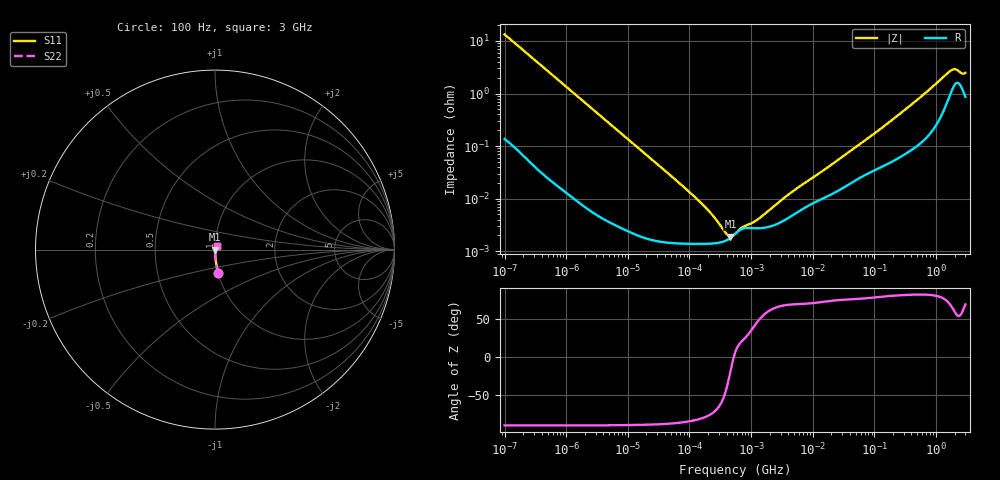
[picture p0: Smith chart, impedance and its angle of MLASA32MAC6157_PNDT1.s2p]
! MLASA32MAC6157_PNDT1  S-PARAMETER MODEL  ( Standard Model )
! Model Generated by TAIYO YUDEN Corporation (http://www.ty-top.com)
! Version 1.0
! TAIYO YUDEN Control No. 220601
! Copyright(c) 2014 TAIYO YUDEN CO.,LTD. All Rights Reserved.
! Product Description (link to TY-COMPAS)
! https://ds.yuden.co.jp/TYCOMPAS/or/detail?pn=MLASA32MAC6157MPNDT1&u=M
! Products Name : Multilayer Ceramic Capacitors
! Characteristics :
!  Capacitance : 150 [uF] , Rated Voltage : 4 [V] , TCC : X6S
!  Case Size : 3.2 x 2.5 / 0.126 x 0.098 [mm/inch] , Thickness : 2.5 / 0.098 [mm/inch]
!  (Conditions: Temperature = 25 [degC] , DC Bias Voltage = 0 [V])
! External Node Assignments :
!  1  o---| |---o  2
! GND o---------o GND
! Frequency Range : 100Hz  -  3GHz  [ 401 STEP ]
# MHZ S RI R 50
! Freq[MHz].  S11 Real  S11 Imag  S21 Real  S21 Imag  S12 Real  S12 Imag  S22 Real  S22 Imag
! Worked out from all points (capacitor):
!   401 points, 100 Hz to 3 GHz, reference 50 ohm
!   read as one part in series: C = 120 uF near 109 Hz
!   lowest |Z| = 1.89 mohm at 461.1 kHz (marker M1)
!   series resonance near 522 kHz, so ESL is about 780 pH
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0.0001  0.0186 -0.1301  0.9814 0.1301  0.9814 0.1301  0.0186 -0.1301
0.000114  0.0146 -0.1149  0.9854 0.1149  0.9854 0.1149  0.0146 -0.1149
0.000175  0.00653 -0.0756  0.9935 0.0756  0.9935 0.0756  0.00653 -0.0756
0.000306  0.00231 -0.0436  0.9977 0.0436  0.9977 0.0436  0.00231 -0.0436
0.001788  0.000133 -0.00755  0.9999 0.00755  0.9999 0.00755  0.000133 -0.00755
0.031977  1.55e-05 -0.000427  1 0.000427  1 0.000427  1.55e-05 -0.000427
0.121426  1.38e-05 -0.000107  1 0.000107  1 0.000107  1.38e-05 -0.000107
0.132342  1.38e-05 -9.74e-05  1 9.74e-05  1 9.74e-05  1.38e-05 -9.74e-05
0.144239  1.38e-05 -8.83e-05  1 8.83e-05  1 8.83e-05  1.38e-05 -8.83e-05
0.461094  1.79e-05 -6.08e-06  1 6.08e-06  1 6.08e-06  1.79e-05 -6.08e-06
0.547723  2.12e-05 2.11e-06  1 -2.11e-06  1 -2.11e-06  2.12e-05 2.11e-06
3.198641  3.68e-05 8.97e-05  1 -8.97e-05  1 -8.97e-05  3.68e-05 8.97e-05
3.639519  4e-05 0.000102  1 -0.000102  1 -0.000102  4e-05 0.000102
9.794414  8.02e-05 0.000234  0.9999 -0.000234  0.9999 -0.000234  8.02e-05 0.000234
22.1892  0.000128 0.000463  0.9999 -0.000463  0.9999 -0.000463  0.000128 0.000463
175.1444  0.000482 0.00282  0.9995 -0.00282  0.9995 -0.00282  0.000482 0.00282
536.3016  0.00115 0.00809  0.9989 -0.00809  0.9989 -0.00809  0.00115 0.00809
1714.41  0.0103 0.0246  0.9897 -0.0246  0.9897 -0.0246  0.0103 0.0246
1868.531  0.0129 0.025  0.9871 -0.025  0.9871 -0.025  0.0129 0.025
2036.508  0.0153 0.0241  0.9847 -0.0241  0.9847 -0.0241  0.0153 0.0241
2636.591  0.0128 0.0201  0.9872 -0.0201  0.9872 -0.0201  0.0128 0.0201
3000  0.00911 0.0227  0.9909 -0.0227  0.9909 -0.0227  0.00911 0.0227
